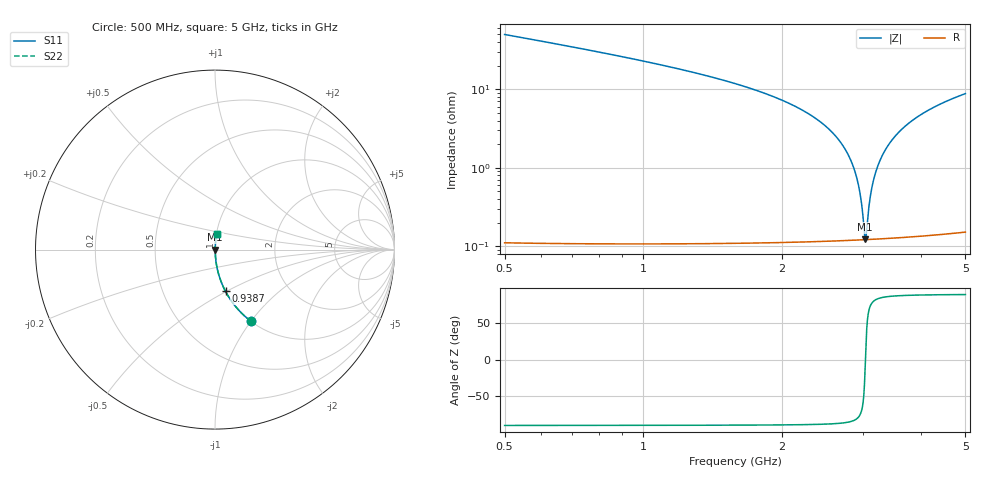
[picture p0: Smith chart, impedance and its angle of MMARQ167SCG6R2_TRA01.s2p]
! MMARQ167SCG6R2_TRA01  S-PARAMETER MODEL  ( General Type )
! Model Generated by TAIYO YUDEN Corporation (http://www.ty-top.com)
! Version 1.0
! TAIYO YUDEN Control No. 160201
! Copyright(c) 2016 TAIYO YUDEN CO.,LTD. All Rights Reserved.
! Product Description (link to TY-COMPAS)
! https://ds.yuden.co.jp/TYCOMPAS/or/detail?pn=MMARQ167SCG6R2CTRA01&u=M
! Products Name : Multilayer Ceramic Capacitors
! Characteristics :
!  Capacitance : 6.2 pF , Rated Voltage : 250V , TCC : CG / C0G
!  Case Size : 1.6 x 0.8 / 0.063 x 0.031 [mm/inch] , Thickness : 0.7 / 0.028 [mm/inch]
!  (Conditions: Temperature = 25 degC , DC Bias Current/Voltage = 0A / 0V)
! External Node Assignments :
!  1  o---| |---o  2
! GND o---------o GND
! Frequency Range : 500MHz  -  5000MHz  [ 401 STEP ]
# MHz S RI R 50
! Freq[MHz].  S11 Real  S11 Imag  S21 Real  S21 Imag  S12 Real  S12 Imag  S22 Real  S22 Imag
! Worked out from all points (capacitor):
!   401 points, 500 MHz to 5 GHz, reference 50 ohm
!   read as one part in series: C = 6.2 pF near 522.5 MHz
!   lowest |Z| = 122 mohm at 3.031 GHz (marker M1)
!   series resonance near 3.034 GHz, so ESL is about 440 pH
!   S11 on the Smith chart (normalised r, x): 500 MHz: 1.00, -1.00; 938.8 MHz: 1.00, -0.49; 5 GHz: 1.00, +0.18
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500  0.2003 -0.3991  0.7997 0.3991  0.7997 0.3991  0.2003 -0.3991
691.25  0.1111 -0.3127  0.8889 0.3127  0.8889 0.3127  0.1111 -0.3127
938.75  0.0585 -0.2326  0.9415 0.2326  0.9415 0.2326  0.0585 -0.2326
1253.75  0.029 -0.1647  0.971 0.1647  0.971 0.1647  0.029 -0.1647
2007.5  0.00624 -0.0714  0.9938 0.0714  0.9938 0.0714  0.00624 -0.0714
2457.5  0.00244 -0.0358  0.9976 0.0358  0.9976 0.0358  0.00244 -0.0358
2626.25  0.00177 -0.0244  0.9982 0.0244  0.9982 0.0244  0.00177 -0.0244
2750  0.00146 -0.0166  0.9985 0.0166  0.9985 0.0166  0.00146 -0.0166
2851.25  0.0013 -0.0105  0.9987 0.0105  0.9987 0.0105  0.0013 -0.0105
2918.75  0.00124 -0.00655  0.9988 0.00655  0.9988 0.00655  0.00124 -0.00655
2963.75  0.00122 -0.00396  0.9988 0.00396  0.9988 0.00396  0.00122 -0.00396
3008.75  0.00121 -0.00142  0.9988 0.00142  0.9988 0.00142  0.00121 -0.00142
3031.25  0.00121 -0.000159  0.9988 0.000159  0.9988 0.000159  0.00121 -0.000159
3053.75  0.00121 0.00109  0.9988 -0.00109  0.9988 -0.00109  0.00121 0.00109
3087.5  0.00122 0.00295  0.9988 -0.00295  0.9988 -0.00295  0.00122 0.00295
3121.25  0.00124 0.00478  0.9988 -0.00478  0.9988 -0.00478  0.00124 0.00478
3200  0.00131 0.00899  0.9987 -0.00899  0.9987 -0.00899  0.00131 0.00899
3323.75  0.00148 0.0154  0.9985 -0.0154  0.9985 -0.0154  0.00148 0.0154
3503.75  0.00186 0.0244  0.9981 -0.0244  0.9981 -0.0244  0.00186 0.0244
3818.75  0.00285 0.0391  0.9972 -0.0391  0.9972 -0.0391  0.00285 0.0391
4257.5  0.00477 0.0581  0.9952 -0.0581  0.9952 -0.0581  0.00477 0.0581
5000  0.00918 0.0872  0.9908 -0.0872  0.9908 -0.0872  0.00918 0.0872
